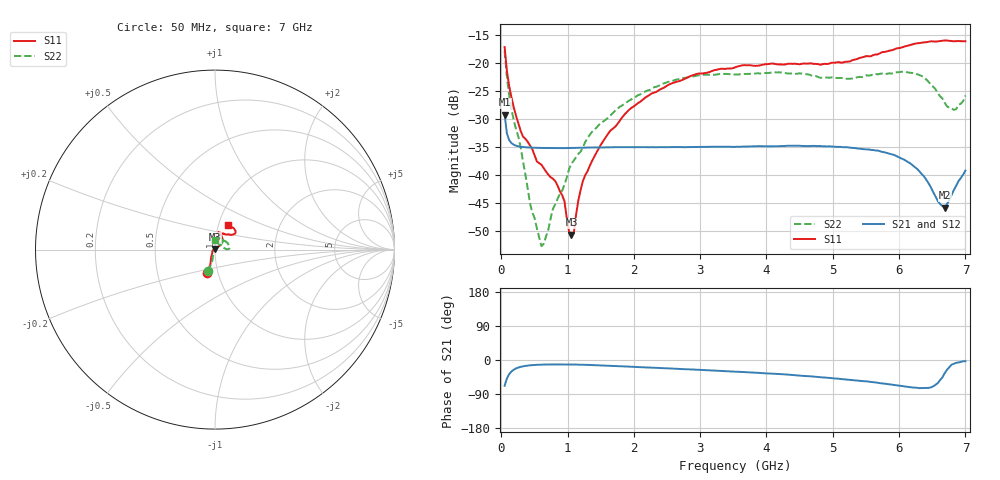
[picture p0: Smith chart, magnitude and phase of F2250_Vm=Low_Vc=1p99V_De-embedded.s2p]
! Integrated Device Technology
! Corporate Headquarters
! 6024 Silver Creek Valley Road
! San Jose, CA 95138  USA
! Phone:  1-408-284-8200
! Toll Free:  1-800-223-1366
! Webpage:  http://www.idt.com/
! Timing and RF Division
! 515 Groton Road, Suite 102
! Westford, MA 01886-6024
! Device:  F2250
! Description: Voltage Variable RF Attenuator
! Frequency:  50.0 -  6000.00 MHz
! Package:  3x3 mm Thin QFN Plastic Package: 16 pin
! Ports:  2 RF, 3 DC
!  Pin  1  = GND
!  Pin  2  = NC
!  Pin  3  = RF1  = Port 1
!  Pin  4  = NC
!  Pin  5  = GND
!  Pin  6  = GND
!  Pin  7  = GND
!  Pin  8  = GND
!  Pin  9  = NC
!  Pin 10  = RF2  = Port 2
!  Pin 11  = NC
!  Pin 12  = GND
!  Pin 13  = GND
!  Pin 14  = VCNTRL
!  Pin 15  = VDD
!  Pin 16  = VMODE
! Vcntrl:  1.990 Volts
! Vmode:  +0.000 Volts
! Vdd:  +3.30  Volts
! Current:  1.182 mA
! Data:  The device was measured on a the F2250 evaluation board which has
!  individual transmission lines to the RF pins.  Data was collected
!  using a calibrated network analyzer.  The evaluation board was
!  de-embedded using a TRL calibration technique.
!  The reference plane is the edge of the package pin.
! Misc:  SN 10
!  Action Tracker AT0258
! Date Measured:  2014-11-26
! Date:  2015-10-15  MJV
! Note:
!  Integrated Device Technology supplies this data as a sample of measured
!  data at the package pin for this product.  Your particular data for this
!  product may vary.
!  Data was taken at 25 degrees C.
!  Integrated Device Technology reserves the right to change this data at anytime.
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# GHz S dB R 50
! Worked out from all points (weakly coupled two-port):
!   201 points, 50 MHz to 7 GHz, reference 50 ohm
!   highest |S21| = -29.25 dB at 50 MHz (marker M1); lowest = -45.9 dB at 6.687 GHz (marker M2)
!   lowest |S11| = -50.7 dB at 1.058 GHz (marker M3), VSWR 1.01, Z = 49.8 + j0.246 ohm
!   |S11| at or under -10 dB: start of sweep to end of sweep
!   |S22| runs from -52.8 to -17.9 dB; largest |S21 - S12| = 5e-05
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0.05  -17.18 -108.6  -29.25 -68.0  -29.25 -68.0  -17.85 -108.1
0.08475  -21.44 -107.4  -32.62 -48.8  -32.62 -48.8  -22.55 -103.1
0.1195  -24.20 -111.7  -33.82 -37.3  -33.82 -37.3  -25.88 -105.4
0.29325  -32.20 -127.5  -35.00 -18.0  -35.00 -18.0  -35.17 -109.0
0.43225  -34.76 -144.6  -35.15 -14.0  -35.15 -14.0  -45.07 -130.8
0.606  -38.23 -160.7  -35.22 -12.2  -35.21 -12.2  -52.78 149.6
0.77975  -40.73 177.7  -35.24 -11.7  -35.24 -11.7  -46.10 81.9
0.91875  -43.67 158.0  -35.25 -11.7  -35.24 -11.7  -42.84 65.2
1.023  -50.25 144.0  -35.24 -11.8  -35.23 -11.9  -38.96 60.3
1.05775  -50.74 121.8  -35.23 -11.9  -35.23 -11.9  -38.02 58.5
1.0925  -50.48 89.4  -35.22 -12.0  -35.22 -12.0  -37.50 54.8
1.162  -44.62 56.1  -35.20 -12.2  -35.20 -12.2  -36.28 47.3
1.2315  -41.10 43.6  -35.18 -12.5  -35.17 -12.5  -35.11 42.6
1.6485  -32.09 41.8  -35.10 -15.2  -35.10 -15.2  -29.39 43.1
2.37825  -24.87 47.3  -35.07 -21.0  -35.07 -21.0  -24.07 45.6
3.525  -20.80 72.4  -35.02 -30.6  -35.02 -30.6  -22.09 68.8
4.7065  -20.17 72.3  -34.85 -43.8  -34.84 -43.8  -22.32 68.8
5.85325  -17.82 40.4  -36.23 -64.2  -36.24 -64.3  -21.87 16.8
6.33975  -16.40 40.9  -39.87 -74.1  -39.87 -74.2  -22.34 2.7
6.68725  -15.99 48.8  -45.88 -34.9  -45.88 -34.6  -27.13 23.0
6.82625  -16.14 53.6  -42.73 -9.9  -42.68 -9.8  -28.41 52.5
7  -16.12 63.2  -39.25 -3.1  -39.22 -3.2  -25.84 87.8
